FUNCTION_BLOCK FB_DO_IED_LD1_LEDGGIO6_SPCSO1 EXTENDS FB_AcsiCommonControllableDataClass
VAR_INPUT
	stVal: FB_AcsiBATypeBOOLEAN := (fc:=ACSI_FC_ST, TrgOp:=ACSI_TrgOp_dchg, bLinkResult:=THIS^.AddDataToContainer(ipData:=stVal));
	q: FB_AcsiDATypeQuality := (fc:=ACSI_FC_ST, TrgOp:=ACSI_TrgOp_qchg, bLinkResult:=THIS^.AddDataToContainer(ipData:=q));
	t: FB_AcsiDATypeTimeStamp := (fc:=ACSI_FC_ST, bLinkResult:=THIS^.AddDataToContainer(ipData:=t));
	stSeld: FB_AcsiBATypeBOOLEAN := (fc:=ACSI_FC_ST, TrgOp:=ACSI_TrgOp_dchg, bLinkResult:=THIS^.AddDataToContainer(ipData:=stSeld));
	ctlModel: FB_AcsiDATypeCtlModels := (fc:=ACSI_FC_CF, TrgOp:=ACSI_TrgOp_dchg, eValue:=E_AcsiCtlModels.DirectWithEnhancedSecurity, bLinkResult:=THIS^.AddDataToContainer(ipData:=ctlModel));
	Oper: FB_AcsiCDC_Oper_BOOLEAN := (fc:=ACSI_FC_CO, bLinkResult:=THIS^.AddDataToContainer(ipData:=Oper));
	
	
	fbControl: FB_DirectControl := (ipCtrl:=THIS^.AddServerJob(ipEvent:=fbControl, ipCompletion:=fbControl), eType:=E_AcsiCDCType.SPC, ipBehVal:=fbIED.IEDLD1.LEDGGIO6.Beh.stVal);
END_VAR
VAR
END_VAR

END_FUNCTION_BLOCK
